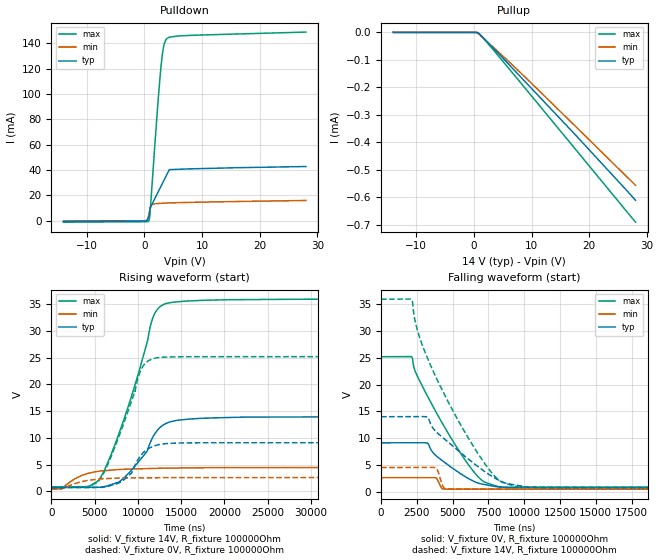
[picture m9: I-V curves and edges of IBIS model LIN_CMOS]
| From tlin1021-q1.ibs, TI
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|   LIN_CMOS Model
[Model]   LIN_CMOS
Model_type   Output
Polarity   Non-Inverting
Vmeas = 7
Vref = 7
Cref = 2pF
Rref = 100000
|   typ   min   max
C_comp   12.71pF   12.14pF   13.31pF
[Voltage Range]   14   4.5   36
[Temperature Range]   25   165   -55
[Pullup Reference]   14   4.5   36
[Pulldown Reference]   0   0   0
[Power Clamp Reference]   14   4.5   36
[GND Clamp Reference]   0   0   0
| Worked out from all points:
|   slope of the pulldown table from 0 to 2.1 V, typ, clamps not added: 104 ohm
|   slope of the pullup table from 0 to 2.1 V, typ, clamps not added: 69.5 kohm
|   falling waveform, V_fixture 0V, R_fixture 100000Ohm: 20-80 % time 2.56us typ, 230ns min, 3.16us max; typ from 9.11 V to 0.708 V
|   rising waveform, V_fixture 14V, R_fixture 100000Ohm: 20-80 % time 3.3us typ, 3.41us min, 4.07us max; typ from 0.724 V to 14 V
|   rising waveform, V_fixture 0V, R_fixture 100000Ohm: 20-80 % time 2.2us typ, 2.96us min, 3.19us max; typ from 0.708 V to 9.11 V
|   falling waveform, V_fixture 14V, R_fixture 100000Ohm: 20-80 % time 3.64us typ, 289ns min, 3.91us max; typ from 14 V to 0.724 V
[Pulldown]
|   Voltage   I(typ)   I(min)   I(max)
-14V      -610.8uA   -360.5uA   -1.256mA
155.1mV   -289.2uA   -72.48uA   -884.7uA
569.8mV   1.346mA    680.1uA    -864.3uA
772.2mV   3.109mA    4.658mA    -277.3uA
964.4mV   8.104mA    8.853mA    4.653mA
1.32V     12.86mA    12.58mA    26.87mA
2.213V    20.98mA    13.42mA    83.98mA
2.887V    27.09mA    13.63mA    121.1mA
3.344V    31.25mA    13.77mA    137.4mA
3.908V    36.38mA    13.89mA    143.7mA
4.331V    40.21mA    13.97mA    144.8mA
28V       42.71mA    15.89mA    148.9mA
[Pullup]
|   Voltage   I(typ)   I(min)   I(max)
-14V      376.4nA    200.2nA    962.6nA
296.6mV   -185.8nA   -244.4nA   -164.2nA
734.8mV   -1.77uA    -4.627uA   -1.828uA
2.887V    -47.45uA   -45.08uA   -51.95uA
8.388V    -168.6uA   -153.2uA   -190.9uA
17.62V    -373.9uA   -342.5uA   -426.1uA
28V       -610.9uA   -556.5uA   -690.7uA
[Ramp]
R_load = 100000
|   typ   min   max
dV/dt_r   7.95411/3.27602e-06   2.41328/3.37575e-06   21.0573/4.06354e-06
dV/dt_f   5.03837/2.54792e-06   1.28892/2.24352e-07   14.6331/3.16395e-06
[Falling Waveform]
V_fixture = 0V
V_fixture_min = 0V
V_fixture_max = 0V
R_fixture = 100000Ohm
C_fixture = 0F
|   Time   V(typ)   V(min)   V(max)
0s        9.105V     2.596V     25.19V
2.149us   9.117V     2.594V     25.15V
2.391us   9.118V     2.593V     22.45V
3.221us   9.067V     2.592V     17.95V
3.863us   6.656V     2.499V     14.76V
4.316us   5.698V     493.1mV    12.62V
5.786us   2.951V     455mV      6.245V
7.015us   1.419V     454.8mV    2.173V
8.244us   861.8mV    454.6mV    906.3mV
50us      708.2mV    448.3mV    802.6mV
[Rising Waveform]
V_fixture = 14V
V_fixture_min = 4.5V
V_fixture_max = 36V
R_fixture = 100000Ohm
C_fixture = 0F
|   Time   V(typ)   V(min)   V(max)
0s        724.4mV    471.5mV    833.6mV
4.176us   768.6mV    3.35V      915.2mV
5.636us   784mV      3.81V      2.502V
6.922us   1.272V     3.979V     6.981V
8.849us   3.268V     4.16V      15.69V
11.05us   7.459V     4.264V     27.76V
11.73us   10.16V     4.296V     32.44V
12.98us   12.46V     4.346V     34.93V
22.24us   13.88V     4.444V     35.83V
50us      13.98V     4.494V     35.93V
[Rising Waveform]
V_fixture = 0V
V_fixture_min = 0V
V_fixture_max = 0V
R_fixture = 100000Ohm
C_fixture = 0F
|   Time   V(typ)   V(min)   V(max)
0s        708.2mV    448.3mV    802.6mV
4.176us   715.8mV    2.048V     858.8mV
5.509us   749.1mV    2.311V     2.029V
6.547us   953.8mV    2.411V     5.151V
8.362us   2.146V     2.512V     12.73V
9.268us   3.426V     2.523V     16.9V
10.31us   6.643V     2.536V     22.54V
11.73us   8.414V     2.553V     24.8V
14.67us   9.044V     2.583V     25.14V
50us      9.105V     2.596V     25.19V
[Falling Waveform]
|Gnd
V_fixture = 14V
V_fixture_min = 4.5V
V_fixture_max = 36V
R_fixture = 100000Ohm
C_fixture = 0F
|   Time   V(typ)   V(min)   V(max)
0s        13.98V     4.494V     35.93V
2.151us   14V        4.504V     35.89V
2.42us    14V        4.505V     31.42V
2.94us    14V        4.508V     26.95V
3.8us     11.33V     4.47V      21.59V
4.404us   9.876V     667.3mV    18.27V
5.256us   7.95V      482.7mV    13.93V
7.793us   2.785V     482mV      3.316V
9.313us   1.258V     481.7mV    1.016V
50us      724.4mV    471.5mV    833.6mV
